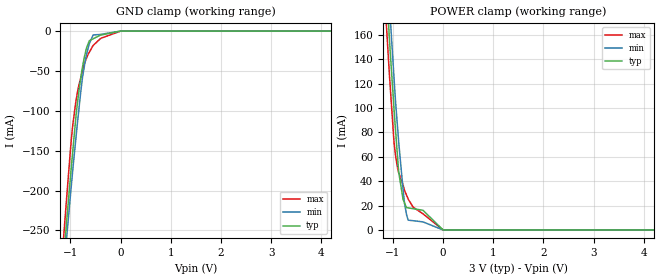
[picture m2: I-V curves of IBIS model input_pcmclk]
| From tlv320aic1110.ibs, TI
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|   input_pcmclk Model
[Model]   input_pcmclk
Model_type   Input
Vinl = 0.9
Vinh = 2.1
|   typ   min   max
|   (nom PVT)   (Fast PVT)   (slow PVT)
|Average
C_comp   2.321e-12   2.321e-12   2.329e-12
| Where nom  PVT is Nominal Process,  3V,  65C
|   Fast PVT is Strong Process,   3.3V,  -40C
|   Slow PVT is Weak Process,   2.7V,  125C
[Model Spec]
|   typ   min   max
Vinl   0.9   0.81   0.99
Vinh   2.1   1.89   2.31
[Voltage Range]   3   2.7   3.3
|Ambient Temperature   25   105   -40
|Junction Temperature
[Temperature Range]   65   125   -40
[Power Clamp Reference]   3   2.7   3.3
[GND Clamp Reference]   0   0   0
[GND Clamp]
-3V       -1.894A    -1.82A     -1.989A
-1.149V   -294.7mA   -311.2mA   -268.7mA
-1.083V   -243.7mA   -263.7mA   -214.3mA
-1.065V   -230.1mA   -251mA     -200.2mA
-980.4mV  -168.8mA   -191.9mA   -133.6mA
-950.7mV  -148mA     -171.6mA   -116.3mA
-882mV    -101.7mA   -128.2mA   -84.57mA
-780mV    -52.8mA    -68.45mA   -54.83mA
-678mV    -20.79mA   -28.69mA   -33.79mA
-548.4mV  -9.673mA   -4.822mA   -18.06mA
-300uV    0A         0A         0A
6V        0A         0A         0A
[POWER Clamp]
-3V       1.735A     1.693A     1.846A
-1.132V   199.6mA    226.4mA    168.5mA
-1.069V   155.7mA    184.1mA    126.4mA
-1.059V   148.6mA    177.2mA    120.1mA
-977.1mV  98.11mA    123.4mA    70.99mA
-885mV    47.39mA    71.74mA    46.95mA
-798.9mV  25.15mA    33.32mA    37.12mA
-769.8mV  22.2mA     21.79mA    32.53mA
-696.6mV  18.12mA    8.037mA    25.3mA
-402.9mV  16.17mA    6.639mA    13.3mA
-300uV    0A         0A         0A
6V        0A         0A         0A
